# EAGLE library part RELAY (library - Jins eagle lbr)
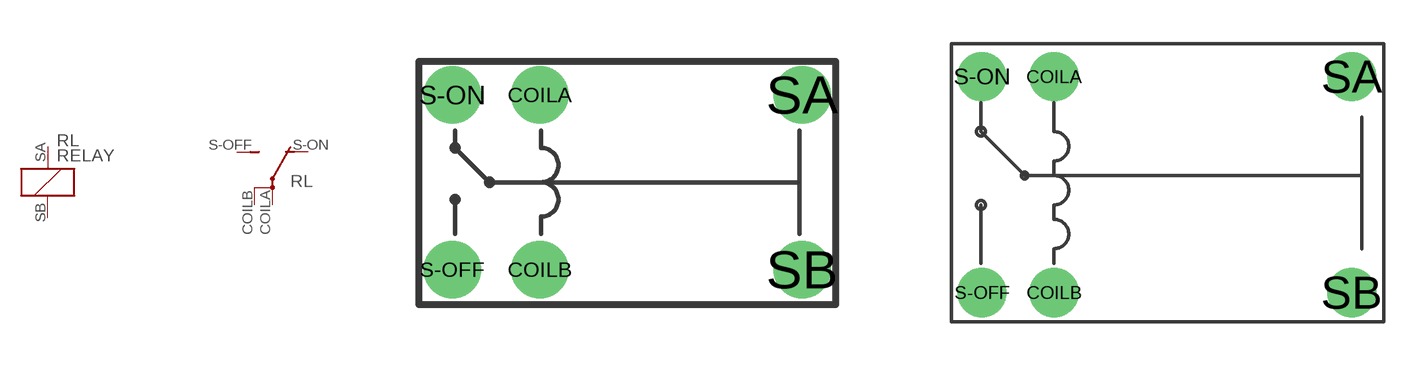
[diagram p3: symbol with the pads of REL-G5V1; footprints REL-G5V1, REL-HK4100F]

Designator prefix RL; gates G$1=REL-4PINS G$2=REL-COIL

## RELAY-1A  [REL-G5V1]
COILA  G$1:P  pas
COILB  G$1:P  pas
S-OFF  G$1:SW  pas
S-ON  G$1:ON  pas
SA  G$2:1  pas
SB  G$2:2  pas

## RELAY-3A  [REL-HK4100F]
Pads as for REL-G5V1

## Footprint REL-G5V1 (pad centres in mm)
drill 0.813 pad 1.676: COILA -2.54,2.54; COILB -2.54,-2.54; S-OFF -5.08,-2.54; S-ON -5.08,2.54; SA 5.08,2.54; SB 5.08,-2.54

## Footprint REL-HK4100F (pad centres in mm)
drill 0.813 pad 1.676: COILA -4,4.38; COILB -4,-3; S-OFF -6.46,-3; S-ON -6.46,4.38; SA 6.16,4.38; SB 6.16,-3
